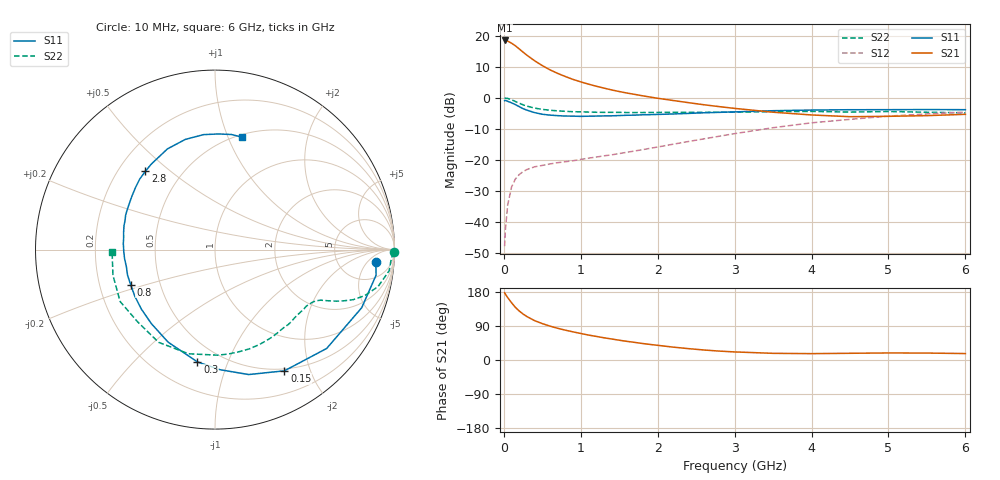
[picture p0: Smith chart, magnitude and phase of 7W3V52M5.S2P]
! Infineon Technologies  Discrete & RF Semiconductors
! BFS17W
! Si NPN RF Bipolar Junction Transistor in SOT323
! VCE = 3.5 V  IC = 2.5 mA
! Common Emitter S-Parameters:  August  1999
# GHz  S  MA  R  50
!  f  S11  S21  S12  S22
! GHz  MAG  ANG  MAG  ANG  MAG  ANG  MAG  ANG
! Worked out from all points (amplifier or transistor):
!   36 points, 10 MHz to 6 GHz, reference 50 ohm
!   highest |S21| = 18.5 dB at 10 MHz (marker M1)
!   |S21| within 3 dB of that: start of sweep to 213.4 MHz
!   unconditionally stable (mu >= 1): 760.2 MHz to 3.229 GHz; 4.032 GHz to end of sweep
!   at 250 MHz: K = 0.40, MSG = 19.2 dB, |S12| = -23.8 dB
!   at 1.4 GHz: K = 1.30, MAG = 7.2 dB, |S12| = -18.4 dB
!   at 6 GHz: K = 1.09, MAG = -2.2 dB, |S12| = -4.6 dB
!   S11 on the Smith chart (normalised r, x): 10 MHz: 13, -9; 150 MHz: 0.47, -1.62; 300 MHz: 0.38, -0.78; 800 MHz: 0.34, -0.18; 2.8 GHz: 0.31, +0.41; 6 GHz: 0.52, +1.12
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0.01  0.8984 -4.3  8.381 177.5  0.0041 80.0  0.998 -0.9
0.02  0.9088 -9.0  8.375 173.9  0.0075 90.1  0.9837 -2.8
0.05  0.8792 -21.6  8.186 164.7  0.0189 79.4  0.9777 -6.9
0.1  0.831 -41.5  7.576 151.2  0.0366 68.7  0.9313 -12.8
0.15  0.7783 -60.2  6.875 138.9  0.0494 60.1  0.8726 -17.1
0.2  0.721 -74.9  6.124 129.3  0.0583 54.1  0.8192 -19.9
0.25  0.6695 -87.7  5.44 121.3  0.0649 49.3  0.772 -21.7
0.3  0.6333 -98.9  4.852 114.6  0.0702 46.3  0.7355 -23.0
0.4  0.5782 -116.8  3.948 103.9  0.0776 43.2  0.6834 -24.6
0.5  0.5441 -130.6  3.301 96.0  0.0817 41.9  0.652 -25.6
0.6  0.5274 -141.1  2.82 89.4  0.0863 42.0  0.6311 -26.9
0.7  0.5167 -149.9  2.473 83.7  0.0904 42.8  0.6172 -28.3
0.8  0.509 -157.5  2.201 78.7  0.0937 44.1  0.6063 -30.2
1.1  0.5066 -174.7  1.662 65.8  0.1069 48.6  0.5904 -36.0
1.3  0.5119 176.3  1.436 58.7  0.1165 51.7  0.5838 -40.8
1.6  0.5243 165.2  1.194 49.2  0.1329 56.4  0.5799 -48.2
2.2  0.5499 147.5  0.906 34.0  0.1792 62.7  0.5839 -64.8
2.8  0.5839 131.7  0.722 23.5  0.241 64.1  0.5864 -82.8
3.5  0.6205 115.3  0.587 17.6  0.3306 60.7  0.5987 -104.2
4.5  0.6438 95.7  0.497 17.7  0.4502 48.9  0.5899 -137.1
5.5  0.6478 81.9  0.517 18.3  0.5505 36.1  0.5863 -165.9
6  0.6444 76.7  0.543 17.0  0.5893 30.0  0.5734 -178.6
